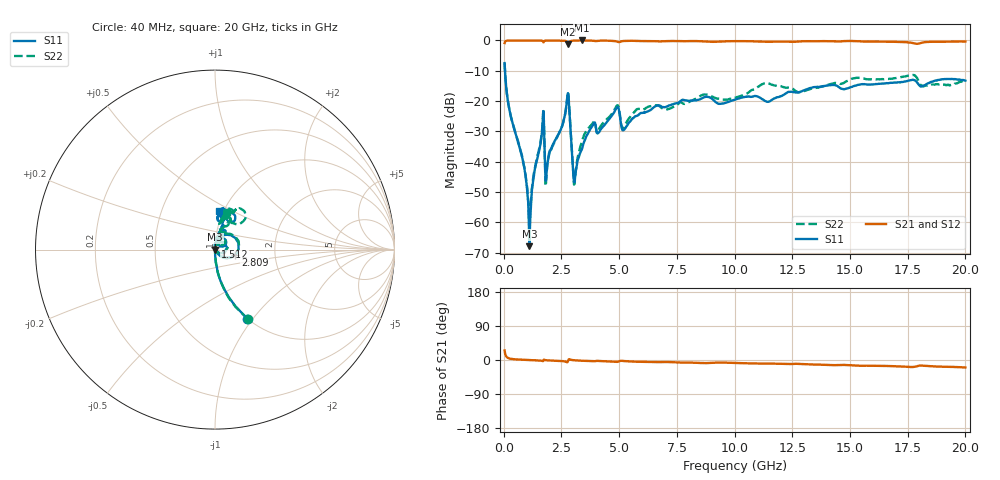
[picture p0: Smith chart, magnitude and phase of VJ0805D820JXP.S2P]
! VJ0805D820JXP
! DATE 10/29/2021  13:35
! CORRECTED  DATA
# GHz  S  MA  R  50.00
!  FREQ  S11M  S11A  S21M  S21A  S12M  S12A  S22M  S22A
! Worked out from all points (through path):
!   1601 points, 40 MHz to 20 GHz, reference 50 ohm
!   highest |S21| = 0.01 dB at 3.383 GHz (marker M1); lowest = -1.3 dB at 2.797 GHz (marker M2)
!   group delay of S21, straight-line fit = 2.86 ps
!   lowest |S11| = -67.9 dB at 1.113 GHz (marker M3), VSWR 1.00, Z = 50 - j0.0202 ohm
!   |S11| at or under -10 dB: 56.32 MHz to end of sweep
!   |S22| runs from -63.4 to -7.4 dB; largest |S21 - S12| = 0.013
!   S11 on the Smith chart (normalised r, x): 40 MHz: 1.00, -0.93; 1.512 GHz: 1.00, +0.03; 2.809 GHz: 1.25, -0.08; 20 GHz: 0.95, +0.43
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0.04  0.4236 -65.0  0.9066 25.1  0.9041 25.1  0.4286 -64.7
0.277025  0.06355 -86.6  0.9976 3.6  0.9979 3.6  0.06461 -86.5
0.86335  0.008832 -87.1  0.9986 0.3  0.9995 0.3  0.009503 -86.9
1.11285  0.0004047 -29.8  0.9984 -0.3  0.9994 -0.3  0.0006864 -31.6
1.51205  0.01423 81.9  0.9967 -1.1  0.9988 -1.2  0.01476 81.1
1.674225  0.03606 70.7  0.9875 -2.4  0.9892 -2.5  0.03788 69.4
1.8863  0.008683 67.0  0.9966 -0.9  0.9975 -0.9  0.009041 74.7
2.796975  0.1312 -0.1  0.8653 -1.0  0.8678 -1.2  0.1353 4.2
2.80945  0.1176 -14.6  0.8817 1.0  0.8828 1.0  0.1212 -10.4
3.05895  0.004939 17.0  0.995 -0.7  0.997 -0.8  0.004246 32.0
3.370825  0.01557 89.6  1 -1.9  1.001 -1.9  0.02041 99.4
3.3833  0.01589 90.4  1.001 -1.9  1.002 -2.1  0.02123 99.7
3.85735  0.03982 81.8  0.9924 -3.0  0.9934 -3.2  0.04308 79.9
4.1318  0.03075 77.1  0.9919 -2.6  0.9946 -2.7  0.03472 83.0
4.8803  0.07623 58.5  0.9669 -5.0  0.9687 -5.2  0.08218 67.6
5.20465  0.03338 50.4  0.9814 -2.7  0.9843 -2.9  0.03672 68.1
6.70165  0.08512 63.2  0.9671 -5.6  0.9685 -5.8  0.08428 64.1
10.02  0.1052 71.6  0.9754 -7.7  0.9766 -8.0  0.1134 74.7
11.35482  0.09935 61.6  0.9547 -9.7  0.9559 -9.9  0.199 69.0
13.35083  0.1675 74.7  0.9733 -11.8  0.9752 -12.2  0.1618 76.5
16.68165  0.1984 77.2  0.9548 -16.0  0.9561 -16.5  0.2328 63.6
20  0.2177 84.7  0.9603 -19.6  0.9625 -20.2  0.2203 71.7
